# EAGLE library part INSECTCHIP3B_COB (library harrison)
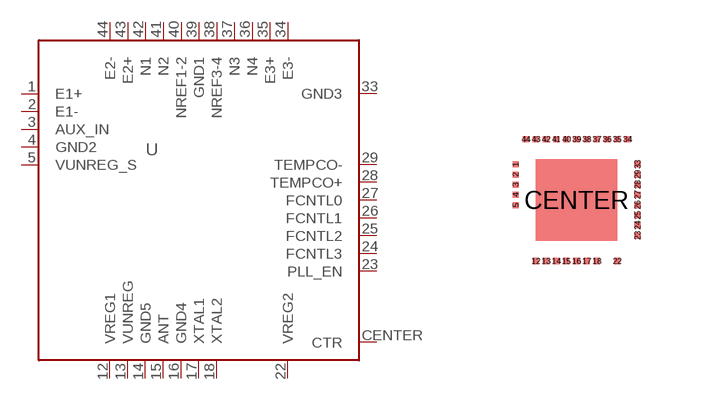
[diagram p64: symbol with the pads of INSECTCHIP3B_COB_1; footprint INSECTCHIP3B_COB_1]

Designator prefix U

## INSECTCHIP3B_COB_1  [INSECTCHIP3B_COB_1]
1  E1+  in
2  E1-  in
3  AUX_IN  in
4  GND2  pwr
5  VUNREG_S  pwr
12  VREG1  pwr
13  VUNREG  pwr
14  GND5  pwr
15  ANT  pas
16  GND4  pwr
17  XTAL1  pas
18  XTAL2  pas
22  VREG2  pwr
23  PLL_EN  in
24  FCNTL3  in
25  FCNTL2  in
26  FCNTL1  in
27  FCNTL0  in
28  TEMPCO+  pas
29  TEMPCO-  pas
33  GND3  pwr
34  E3-  in
35  E3+  in
36  N4  in
37  N3  in
38  NREF3-4  in
39  GND1  pwr
40  NREF1-2  in
41  N2  in
42  N1  in
43  E2+  in
44  E2-  in
CENTER  CTR  pwr

## Footprint INSECTCHIP3B_COB_1 (pad centres in mm)
smd 0.152 x 0.152: 1 -1.524,0.889; 2 -1.524,0.635; 3 -1.524,0.381; 4 -1.524,0.127; 5 -1.524,-0.127; 12 -1.016,-1.524; 13 -0.762,-1.524; 14 -0.508,-1.524; 15 -0.254,-1.524; 16 0,-1.524; 17 0.254,-1.524; 18 0.508,-1.524; 22 1.016,-1.524; 23 1.524,-0.889; 24 1.524,-0.635; 25 1.524,-0.381; 26 1.524,-0.127; 27 1.524,0.127; 28 1.524,0.381; 29 1.524,0.635; 33 1.524,0.889; 34 1.27,1.524; 35 1.016,1.524; 36 0.762,1.524; 37 0.508,1.524; 38 0.254,1.524; 39 0,1.524; 40 -0.254,1.524; 41 -0.508,1.524; 42 -0.762,1.524; 43 -1.016,1.524; 44 -1.27,1.524
smd 2.032 x 2.032: CENTER 0,0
